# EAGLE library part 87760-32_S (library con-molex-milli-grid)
HEADER
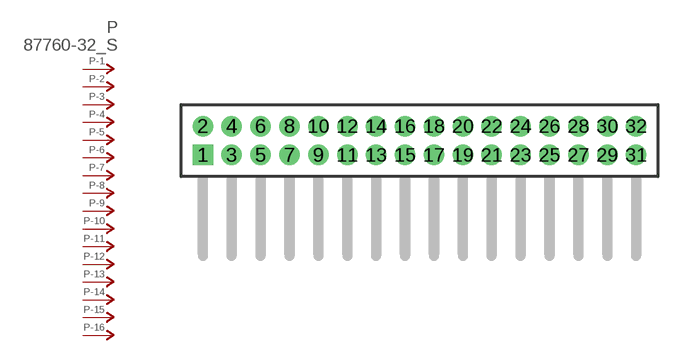
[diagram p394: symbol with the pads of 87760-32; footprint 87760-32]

Designator prefix P; gates -1=P-NV -2=P-N -3=P-N -4=P-N -5=P-N -6=P-N -7=P-N -8=P-N -9=P-N -10=P-N -11=P-N -12=P-N -13=P-N -14=P-N -15=P-N -16=P-N -17=P-N -18=P-N -19=P-N -20=P-N -21=P-N -22=P-N -23=P-N -24=P-N -25=P-N -26=P-N -27=P-N -28=P-N -29=P-N -30=P-N -31=P-N -32=P-N

## 87760-32_S  [87760-32]
1  -1:P  pas
2  -2:P  pas
3  -3:P  pas
4  -4:P  pas
5  -5:P  pas
6  -6:P  pas
7  -7:P  pas
8  -8:P  pas
9  -9:P  pas
10  -10:P  pas
11  -11:P  pas
12  -12:P  pas
13  -13:P  pas
14  -14:P  pas
15  -15:P  pas
16  -16:P  pas
17  -17:P  pas
18  -18:P  pas
19  -19:P  pas
20  -20:P  pas
21  -21:P  pas
22  -22:P  pas
23  -23:P  pas
24  -24:P  pas
25  -25:P  pas
26  -26:P  pas
27  -27:P  pas
28  -28:P  pas
29  -29:P  pas
30  -30:P  pas
31  -31:P  pas
32  -32:P  pas

## Footprint 87760-32 (pad centres in mm)
HEADER Dual Row, Right Angle
drill 0.914 square: 1 -15,-1
drill 0.914: 2 -15,1; 3 -13,-1; 4 -13,1; 5 -11,-1; 6 -11,1; 7 -9,-1; 8 -9,1; 9 -7,-1; 10 -7,1; 11 -5,-1; 12 -5,1; 13 -3,-1; 14 -3,1; 15 -1,-1; 16 -1,1; 17 1,-1; 18 1,1; 19 3,-1; 20 3,1; 21 5,-1; 22 5,1; 23 7,-1; 24 7,1; 25 9,-1; 26 9,1; 27 11,-1; 28 11,1; 29 13,-1; 30 13,1; 31 15,-1; 32 15,1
